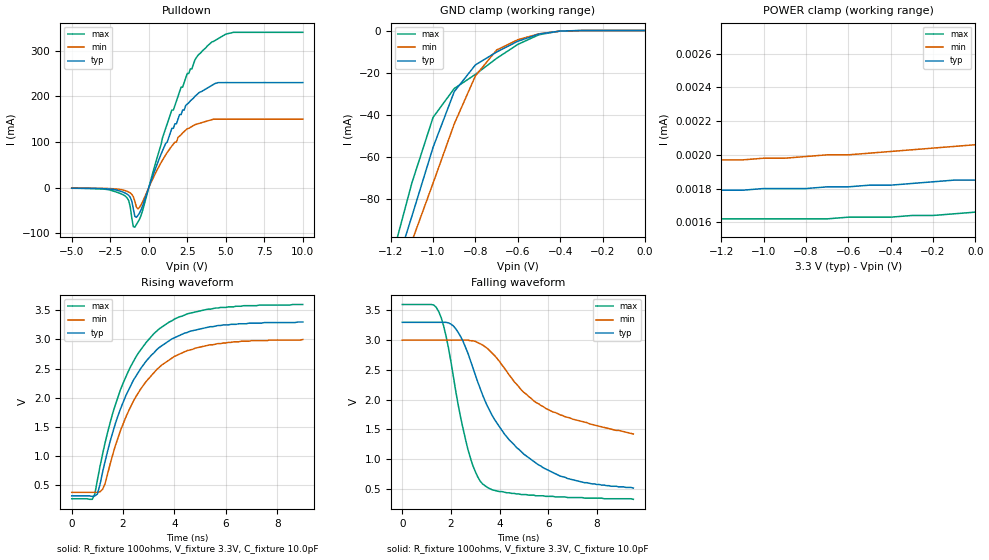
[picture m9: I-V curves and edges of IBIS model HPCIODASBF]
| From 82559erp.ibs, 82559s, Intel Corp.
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[Model]   HPCIODASBF
Model_type   I/O_open_drain
Vinl  =   1.08V   | note : 0.3 * VCCmax
Vinh  =   1.5V   | note : 0.5 * VCCmin
|   typ   min   max
C_comp   2.7pF   NA   NA
|note : on die power/gnd supply distribution R/L/C
|   are not included in the simulation
| note : pull up  mos are not active  pup#="1"
| note : POWER_clamp ref = VIO = VREF = 5.0V
|variable   typ   min   max
[Voltage range]   3.3V   3.0V   3.6V
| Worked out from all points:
|   slope of the pulldown table from 0 to 0.495 V, typ, clamps not added: 10.5 ohm
|   GND clamp passes 1 mA (typ) near -0.45 V on its own axis
|   POWER clamp passes 1 mA (typ) near -2.33 V on its own axis
|   rising waveform, R_fixture 100ohms, V_fixture 3.3V, C_fixture 10.0pF: 20-80 % time 1.74ns typ, 1.77ns min, 1.72ns max; typ from 0.32 V to 3.3 V
|   falling waveform, R_fixture 100ohms, V_fixture 3.3V, C_fixture 10.0pF: 20-80 % time 2.31ns typ, 2.63ns min, 971ps max; typ from 3.3 V to 0.51 V
| note : all DC curves are with 0.2 OHM res. in series to the PAD.
[GND_clamp]
|Voltage  I(typ)   I(min)   I(max)
-5V       -1.63A     -1.47A     -1.85A
-1.2V     -120mA     -130mA     -110mA
-1.1V     -88.1mA    -100mA     -72.3mA
-1V       -55.4mA    -72.4mA    -41.2mA
-900mV    -29mA      -44.3mA    -27.5mA
-800mV    -16.3mA    -21.5mA    -20.8mA
-700mV    -10.2mA    -9.25mA    -13.2mA
-600mV    -5.09mA    -4.37mA    -6.59mA
-500mV    -1.66mA    -1.56mA    -2mA
-400mV    -250uA     -300uA     -220uA
0V        0A         0A         0A
[PullDown]
|Voltage   I(typ)   I(min)   I(max)
-5V       -910uA     -660uA     -1.14mA
-1.6V     -10.6mA    -5.58mA    -16.6mA
-1.2V     -20.9mA    -11.4mA    -41.7mA
-1V       -46.3mA    -19.5mA    -85.1mA
-900mV    -62.5mA    -29.9mA    -86.2mA
-600mV    -55.3mA    -42.9mA    -68.9mA
1.5V      130mA      91.3mA     170mA
2.4V      180mA      126mA      240mA
3.2V      206mA      140mA      290mA
4.3V      228mA      150mA      322mA
5.5V      230mA      150mA      340mA
10V       230mA      150mA      340mA
[POWER_clamp]
|Voltage  I(typ)   I(min)   I(max)
-5V       11.7A      10.4A      13A
-2.4V     3.43mA     5.3uA      460mA
-2.3V     100uA      2.16uA     150mA
-2.2V     4.62uA     2.01uA     10mA
-2.1V     1.9uA      1.99uA     170uA
-2V       1.82uA     1.99uA     4.07uA
-1.9V     1.81uA     1.98uA     1.68uA
-1.8V     1.8uA      1.97uA     1.64uA
-1.4V     1.79uA     1.97uA     1.62uA
-900mV    1.8uA      1.98uA     1.62uA
-400mV    1.82uA     2.02uA     1.63uA
0V        1.85uA     2.06uA     1.66uA
[Ramp]
| note : pad parasitics are not included
|Variable   typ   min   max
dV/dt_r   1.8/0.4n   1.6/0.4n   2.0/0.3n
dV/dt_f   1.7/1.8n   1.0/2.6n   2.0/0.5n
| note : 100ohms RES. always connected to VCC
R_load =   100ohms
[Rising Waveform]
| note : pad parasitics are not included
| note : input changes at T=0.5nS
| note : input data is to vox_data
R_fixture   = 100ohms
V_fixture   = 3.3V
V_fixture_min   = 3.0V
V_fixture_max   = 3.6V
C_fixture   = 10.0pF
| note : the 100ohms RES. is connected to VCC
|Time   typ   min   max
0s        320mV      380mV      270mV
800ps     310mV      380mV      260mV
1ns       350mV      380mV      590mV
1.3ns     910mV      530mV      1.23V
2ns       1.92V      1.55V      2.25V
2.7ns     2.51V      2.16V      2.83V
3.4ns     2.86V      2.52V      3.18V
4.5ns     3.12V      2.81V      3.44V
5.4ns     3.22V      2.91V      3.52V
9ns       3.3V       3V         3.6V
[Falling Waveform]
| note : pad parasitics are not included
| note : input changes at T=0.5nS
| note : input data is to vox_data
R_fixture   = 100ohms
V_fixture   = 3.3V
V_fixture_min   = 3.0V
V_fixture_max   = 3.6V
C_fixture   = 10.0pF
|Time   typ   min   max
0s        3.3V       3V         3.6V
1.5ns     3.3V       3V         3.48V
1.8ns     3.3V       3V         3.07V
2.1ns     3.24V      3V         2.39V
2.7ns     2.78V      3V         1.16V
3.3ns     2.08V      2.92V      580mV
4.2ns     1.42V      2.53V      440mV
5.6ns     900mV      1.93V      380mV
6.8ns     670mV      1.7V       350mV
9.5ns     510mV      1.42V      320mV
